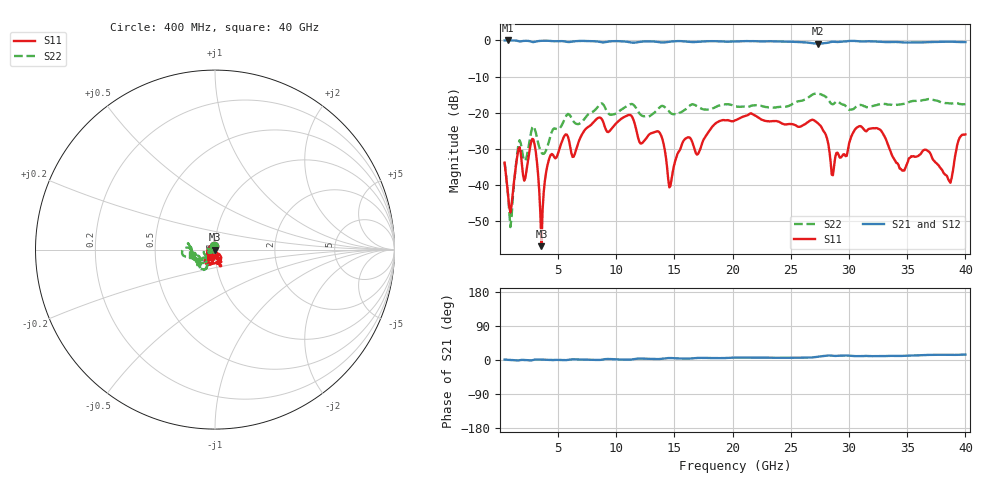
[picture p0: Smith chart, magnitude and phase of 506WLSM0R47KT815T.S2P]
!  American Technical Ceramics  Date:  8/31/2012
!  One Norden Lane
!  Huntington Station,  NY.  11746-2102
!  Tel:  (631) 622-4700  Fax:  (631) 622-4748
!  Part Number  506WLSM0R47KT815T
!  Description:  Ultra-Broadband Inductor
!  Application:  Ultra-broadband DC block decoupling, bias tee
# GHZ S DB R 50
! Freq  |S11|  S11 Ph  |S21|  S21 Ph  |S12|  S12 Ph  |S22|  S22 Ph
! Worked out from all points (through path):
!   401 points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, 400 MHz to 40 GHz, reference 50 ohm
!   highest |S21| = -0.01 dB at 697 MHz (marker M1); lowest = -0.9 dB at 27.33 GHz (marker M2)
!   lowest |S11| = -56.8 dB at 3.568 GHz (marker M3), VSWR 1.00, Z = 49.9 - j0.0846 ohm
!   |S11| at or under -10 dB: start of sweep to end of sweep
!   |S22| runs from -51.6 to -14.7 dB; largest |S21 - S12| = 0.006
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0.4  -33.75 103.1  -0.01 1.2  -0.02 1.2  -33.69 99.3
0.697  -42.62 123.4  -0.01 0.4  -0.01 0.5  -42.74 111.5
0.994  -45.61 -147.3  -0.01 -0.0  -0.02 -0.0  -49.07 -137.7
1.588  -30.05 -143.1  -0.20 -1.2  -0.20 -1.2  -28.72 -127.3
2.182  -37.99 -142.4  -0.11 -0.1  -0.12 -0.1  -33.25 -150.2
2.776  -27.19 -162.5  -0.42 -0.7  -0.42 -0.6  -24.07 -149.7
3.568  -56.84 -143.9  -0.11 1.0  -0.11 1.0  -30.99 -171.6
4.36  -31.64 -107.2  -0.15 -0.2  -0.15 -0.2  -26.21 -125.5
7.033  -26.07 -94.4  -0.14 1.1  -0.13 1.1  -22.49 -122.8
11.092  -20.57 -117.2  -0.46 0.9  -0.45 0.9  -17.80 -122.2
12.082  -28.48 -121.1  -0.36 3.8  -0.35 3.9  -20.48 -141.4
13.666  -25.26 -121.9  -0.46 2.5  -0.45 2.5  -18.67 -138.8
14.656  -40.13 -89.7  -0.32 5.1  -0.31 5.0  -20.05 -160.1
15.943  -27.12 -78.9  -0.28 3.6  -0.27 3.6  -19.07 -147.4
20.2  -22.08 -75.1  -0.25 6.3  -0.23 6.2  -18.15 -138.3
26.833  -21.89 -104.7  -0.77 6.7  -0.76 6.5  -15.03 -168.6
27.328  -22.88 -128.3  -0.88 8.6  -0.88 8.5  -14.71 -175.9
28.615  -37.23 -114.5  -0.36 11.2  -0.35 11.0  -17.65 -175.0
30.793  -23.85 -59.9  -0.22 10.1  -0.22 10.0  -18.02 -153.7
33.466  -29.83 -88.5  -0.45 10.8  -0.45 10.6  -17.75 -170.1
38.614  -38.86 -150.6  -0.33 13.7  -0.34 13.5  -17.39 -178.4
40  -25.97 -123.1  -0.46 14.3  -0.47 14.0  -17.59 -167.4
